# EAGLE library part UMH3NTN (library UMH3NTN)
Bipolar Transistors - Pre-Biased DUAL NPN 50V 100MA SOT-363 Source: Datasheet
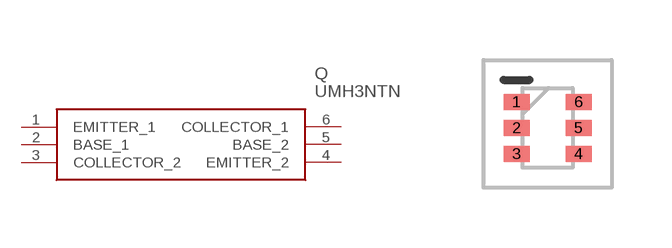
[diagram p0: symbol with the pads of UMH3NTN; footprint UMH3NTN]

Designator prefix Q

## UMH3NTN (Arrow_Part_Number: UMH3NTN; Arrow_Price-Stock: https://www.arrow.com/en/products/umh3ntn/rohm-semiconductor?region=nac; Description: Bipolar Transistors - Pre-Biased DUAL NPN 50V 100MA SOT-363; Height: 1mm; Manufacturer_Name: ROHM Semiconductor; Manufacturer_Part_Number: UMH3NTN; Mouser_Part_Number: 755-UMH3NTN; Mouser_Price-Stock: https://www.mouser.co.uk/ProductDetail/ROHM-Semiconductor/UMH3NTN?qs=4kLU8WoGk0st6ahJ6z2bmw%3D%3D)  [UMH3NTN]
1  EMITTER_1
2  BASE_1
3  COLLECTOR_2
4  EMITTER_2
5  BASE_2
6  COLLECTOR_1

## Footprint UMH3NTN (pad centres in mm)
UMT6
smd 0.65 x 0.4: 1 -0.775,0.65; 2 -0.775,0; 3 -0.775,-0.65; 4 0.775,-0.65; 5 0.775,0; 6 0.775,0.65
